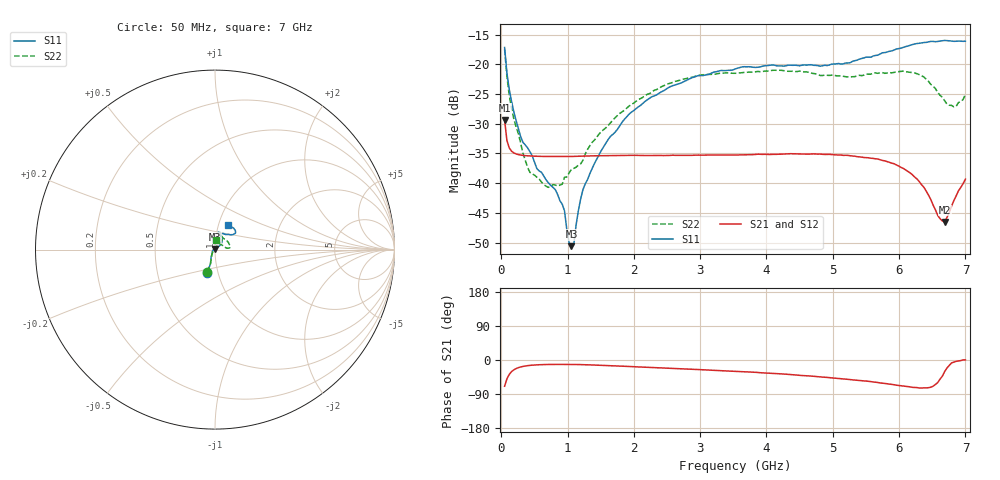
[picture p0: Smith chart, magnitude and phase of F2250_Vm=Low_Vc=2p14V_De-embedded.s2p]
! Integrated Device Technology
! Corporate Headquarters
! 6024 Silver Creek Valley Road
! San Jose, CA 95138  USA
! Phone:  1-408-284-8200
! Toll Free:  1-800-223-1366
! Webpage:  http://www.idt.com/
! Timing and RF Division
! 515 Groton Road, Suite 102
! Westford, MA 01886-6024
! Device:  F2250
! Description: Voltage Variable RF Attenuator
! Frequency:  50.0 -  6000.00 MHz
! Package:  3x3 mm Thin QFN Plastic Package: 16 pin
! Ports:  2 RF, 3 DC
!  Pin  1  = GND
!  Pin  2  = NC
!  Pin  3  = RF1  = Port 1
!  Pin  4  = NC
!  Pin  5  = GND
!  Pin  6  = GND
!  Pin  7  = GND
!  Pin  8  = GND
!  Pin  9  = NC
!  Pin 10  = RF2  = Port 2
!  Pin 11  = NC
!  Pin 12  = GND
!  Pin 13  = GND
!  Pin 14  = VCNTRL
!  Pin 15  = VDD
!  Pin 16  = VMODE
! Vcntrl:  2.140 Volts
! Vmode:  +0.000 Volts
! Vdd:  +3.30  Volts
! Current:  1.179 mA
! Data:  The device was measured on a the F2250 evaluation board which has
!  individual transmission lines to the RF pins.  Data was collected
!  using a calibrated network analyzer.  The evaluation board was
!  de-embedded using a TRL calibration technique.
!  The reference plane is the edge of the package pin.
! Misc:  SN 10
!  Action Tracker AT0258
! Date Measured:  2014-11-26
! Date:  2015-10-15  MJV
! Note:
!  Integrated Device Technology supplies this data as a sample of measured
!  data at the package pin for this product.  Your particular data for this
!  product may vary.
!  Data was taken at 25 degrees C.
!  Integrated Device Technology reserves the right to change this data at anytime.
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# GHz S dB R 50
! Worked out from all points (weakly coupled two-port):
!   201 points, 50 MHz to 7 GHz, reference 50 ohm
!   highest |S21| = -29.36 dB at 50 MHz (marker M1); lowest = -46.5 dB at 6.687 GHz (marker M2)
!   lowest |S11| = -50.6 dB at 1.058 GHz (marker M3), VSWR 1.01, Z = 49.8 + j0.246 ohm
!   |S11| at or under -10 dB: start of sweep to end of sweep
!   |S22| runs from -40.7 to -17.5 dB; largest |S21 - S12| = 5.4e-05
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0.05  -17.18 -108.6  -29.36 -69.2  -29.36 -69.2  -17.48 -110.0
0.08475  -21.45 -107.4  -32.82 -49.8  -32.81 -49.8  -22.05 -107.8
0.189  -28.00 -119.7  -34.91 -26.0  -34.91 -25.9  -29.20 -121.3
0.29325  -32.21 -127.7  -35.28 -18.3  -35.28 -18.3  -33.32 -129.5
0.43225  -34.71 -144.5  -35.43 -14.2  -35.43 -14.2  -38.19 -162.2
0.71025  -39.94 -168.6  -35.52 -11.8  -35.52 -11.8  -40.71 149.7
0.91875  -43.53 158.1  -35.53 -11.6  -35.53 -11.6  -40.18 119.1
0.9535  -44.66 170.1  -35.53 -11.6  -35.53 -11.6  -39.01 118.1
1.023  -49.99 144.4  -35.52 -11.7  -35.52 -11.7  -38.28 100.0
1.05775  -50.61 123.3  -35.51 -11.7  -35.51 -11.7  -37.68 94.9
1.0925  -50.42 88.9  -35.50 -11.8  -35.50 -11.8  -37.53 89.8
1.162  -44.66 56.6  -35.48 -12.0  -35.49 -12.0  -36.97 78.6
1.2315  -41.09 44.4  -35.45 -12.2  -35.46 -12.2  -36.14 69.6
1.6485  -32.11 42.0  -35.37 -14.8  -35.37 -14.8  -29.84 56.6
2.37825  -24.87 47.4  -35.33 -20.5  -35.33 -20.6  -24.06 52.8
3.525  -20.81 72.5  -35.27 -29.9  -35.27 -29.9  -21.52 72.8
4.7065  -20.16 72.3  -35.07 -43.0  -35.07 -42.9  -21.55 71.2
5.85325  -17.82 40.5  -36.49 -63.5  -36.50 -63.6  -21.39 20.9
6.33975  -16.40 41.0  -40.27 -73.8  -40.27 -73.7  -21.91 6.7
6.68725  -15.99 48.8  -46.52 -30.5  -46.51 -30.2  -26.14 26.7
6.861  -16.12 55.1  -42.14 -3.5  -42.08 -3.4  -27.06 58.1
7  -16.12 63.3  -39.33 0.2  -39.30 0.1  -25.04 84.6
